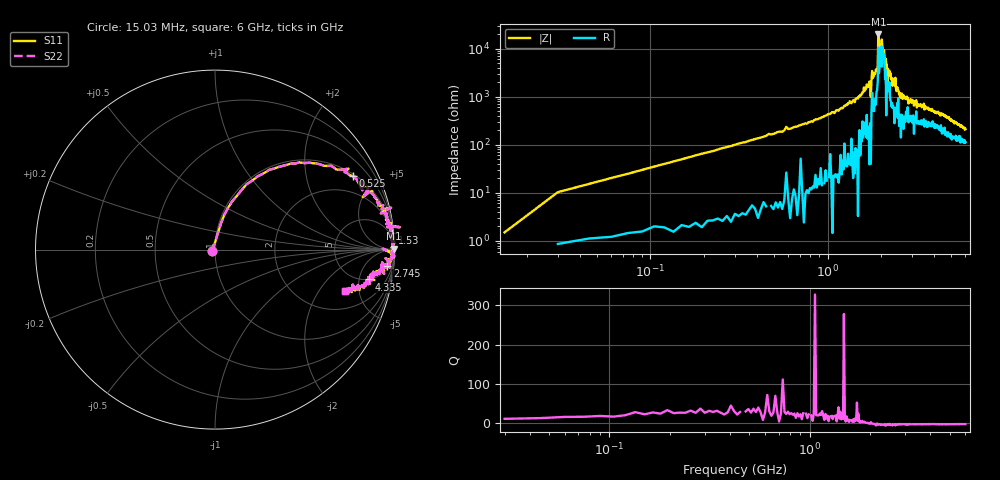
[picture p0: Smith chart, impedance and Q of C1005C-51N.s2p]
!	Network	Analyzer	HP8753E.07.74:	Oct	30	2002	Serial	No.	JP38451487
!	Hewlett-Packard
!	7	Sep	2009	9:10:34
!	Frequency	S11	S21	S12	S22
#	HZ	S	RI	R	50
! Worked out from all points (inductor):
!   400 points, 15.03 MHz to 6 GHz, reference 50 ohm
!   read as one part in series: L = 53.6 nH near 45.03 MHz
!   highest |Z| = 19.6 kohm at 1.935 GHz (marker M1)
!   self-resonance near 1.98 GHz
!   S11 on the Smith chart (normalised r, x): 15.03 MHz: 0.97, -0.02; 525 MHz: 1.10, +3.70; 1.53 GHz: 2, +22; 2.745 GHz: 7, -18; 4.335 GHz: 4.94, -7.04; 6 GHz: 3.25, -3.58
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1.502992e7  -0.0145 -0.00914  1.01 0.00914  1.01 0.00914  -0.0145 -0.00914
3.002985e7  0.0185 0.0999  0.981 -0.0999  0.981 -0.0999  0.0185 0.0999
1.050295e8  0.123 0.301  0.877 -0.301  0.877 -0.301  0.123 0.301
5.250274e8  0.768 0.409  0.232 -0.409  0.232 -0.409  0.768 0.409
1.020025e9  0.94 0.214  0.0598 -0.214  0.0598 -0.214  0.94 0.214
1.530022e9  0.987 0.0909  0.0135 -0.0909  0.0135 -0.0909  0.987 0.0909
1.725021e9  0.997 0.0481  0.00323 -0.0481  0.00323 -0.0481  0.997 0.0481
1.755021e9  0.986 0.0997  0.0142 -0.0997  0.0142 -0.0997  0.986 0.0997
1.785021e9  0.989 0.0269  0.011 -0.0269  0.011 -0.0269  0.989 0.0269
1.92002e9  0.989 0.0196  0.0107 -0.0196  0.0107 -0.0196  0.989 0.0196
1.93502e9  0.997 0.0043  0.00272 -0.0043  0.00272 -0.0043  0.997 0.0043
1.96502e9  0.983 0.0111  0.017 -0.0111  0.017 -0.0111  0.983 0.0111
2.01002e9  0.993 0.00385  0.00684 -0.00385  0.00684 -0.00385  0.993 0.00385
2.160019e9  0.988 -0.0174  0.012 0.0174  0.012 0.0174  0.988 -0.0174
2.175019e9  0.935 0.00513  0.0652 -0.00513  0.0652 -0.00513  0.935 0.00513
2.190019e9  0.987 -0.0228  0.0127 0.0228  0.0127 0.0228  0.987 -0.0228
2.745016e9  0.96 -0.0926  0.0403 0.0926  0.0403 0.0926  0.96 -0.0926
3.015015e9  0.952 -0.101  0.0481 0.101  0.0481 0.101  0.952 -0.101
4.00501e9  0.886 -0.149  0.114 0.149  0.114 0.149  0.886 -0.149
4.335008e9  0.86 -0.166  0.14 0.166  0.14 0.166  0.86 -0.166
5.010005e9  0.828 -0.199  0.172 0.199  0.172 0.199  0.828 -0.199
6e9  0.725 -0.232  0.275 0.232  0.275 0.232  0.725 -0.232
